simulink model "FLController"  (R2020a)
settings: Solver=VariableStepAuto  StartTime=0.0  StopTime=10  RelTol=1e-3
InitFcn:
  | initParams
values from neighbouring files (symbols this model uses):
  K1 = 100    [initParams.m]
  K2 = 100    [initParams.m]
  x0 = [1;1;1]    [initParams.m]

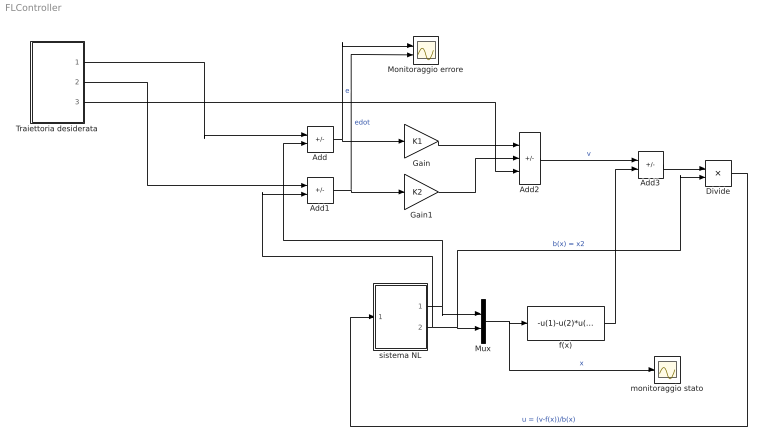
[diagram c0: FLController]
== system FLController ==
  Add : Sum  Inputs=-+
  Add1 : Sum  Inputs=-+
  Add2 : Sum  Inputs=--+
  Add3 : Sum  Inputs=+-
  Divide : Product  Inputs=*/
  Gain : Gain  Gain=K1
  Gain1 : Gain  Gain=K2
  Monitoraggio errore : Scope  NumInputPorts=2
  Mux : Mux  Inputs=2
  Traiettoria desiderata : Subsystem
  f(x) : Fcn  Expr=-u(1)-u(2)*u(2)
  monitoraggio stato : Scope
  sistema NL : Subsystem
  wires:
  Traiettoria desiderata/1(x_d) -> Add/1
  sistema NL/1(x1) -> Add/2, Mux/1
  sistema NL/2(x2) -> Add1/2, Divide/2, Mux/2  "b(x) = x2"
  Add/1 -> Monitoraggio errore/1, Gain/1  "e"
  Add1/1 -> Monitoraggio errore/2, Gain1/1  "edot"
  Gain/1 -> Add2/1
  Gain1/1 -> Add2/2
  Add2/1 -> Add3/1  "v"
  Mux/1 -> monitoraggio stato/1, f(x)/1  "x"
  f(x)/1 -> Add3/2
  Add3/1 -> Divide/1
  Divide/1 -> sistema NL/1(u)  "u = (v-f(x))/b(x)"
  Traiettoria desiderata/2(xdot_d) -> Add1/1
  Traiettoria desiderata/3(xddot_d) -> Add2/3

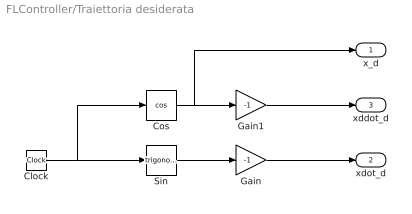
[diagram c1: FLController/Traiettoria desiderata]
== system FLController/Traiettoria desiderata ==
  Clock : Clock
  Cos : Trigonometry  Operator=cos
  Gain : Gain  Gain=-1
  Gain1 : Gain  Gain=-1
  Sin : Trigonometry
  x_d : Outport
  xdot_d : Outport  Port=2
  xddot_d : Outport  Port=3
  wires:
  Clock/1 -> Cos/1, Sin/1
  Sin/1 -> Gain/1
  Cos/1 -> x_d/1, Gain1/1
  Gain1/1 -> xddot_d/1
  Gain/1 -> xdot_d/1

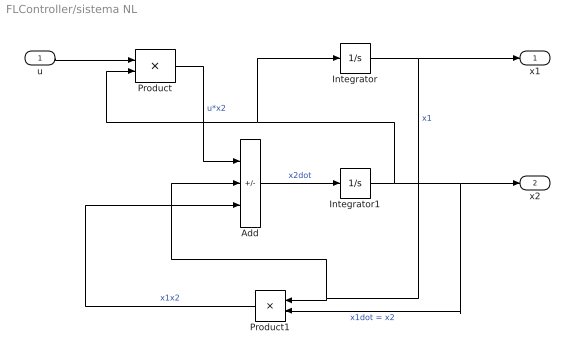
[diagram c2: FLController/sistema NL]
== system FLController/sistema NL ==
  u : Inport
  Add : Sum  Inputs=+--
  Integrator : Integrator  InitialCondition=x0(1)
  Integrator1 : Integrator  InitialCondition=x0(2)  UpperSaturationLimit=100  LowerSaturationLimit=-100
  Product : Product
  Product1 : Product
  x1 : Outport
  x2 : Outport  Port=2
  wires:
  Product/1 -> Add/1  "u*x2"
  Integrator/1 -> Add/2, Product1/1, x1/1  "x1"
  Integrator1/1 -> Integrator/1, Product/2, x2/1, Product1/2  "x1dot = x2"
  u/1 -> Product/1
  Add/1 -> Integrator1/1  "x2dot"
  Product1/1 -> Add/3  "x1x2"
